[IBIS Ver]   3.2
[File Name]   sprm432.ibs
[File Rev]   1.0
[Date]   November 3, 2003
[Source]   File originated at Texas Instruments
[Copyright]   (c) 2003, Texas Instruments Inc.
[Component]   f28235zhh
[Manufacturer] Texas Instruments
[Package]
| Variable   Typ   Min   Max
R_pkg   0.08821   0.00445   0.1444
L_pkg   2.312e-09   3.373e-10   3.933e-09
C_pkg   2.855e-13   1.279e-13   4.259e-13
[Pin] signal_name   model_name   R_pin   L_pin   C_pin
B2   GPIO[30]   BC3325CFHYPU  0.09209  2.36e-09   2.324e-13
C2   GPIO[29]   BC3325CFHYPU  0.08702  2.145e-09  2.491e-13
C3   VSS   NC   0.08455  2.129e-09  2.412e-13
B1   VDD   NC   0.1237   3.291e-09  3.802e-13
C1   GPIO[0]   BC3350AFHYPU  0.103   2.673e-09  3.339e-13
D3   GPIO[1]   BC3350AFHYPU  0.07884  2.005e-09  2.389e-13
D2   GPIO[2]   BC3350AFHYPU  0.07849  1.946e-09  2.548e-13
D1   VSS   NC   0.09972  2.597e-09  2.918e-13
F5   VDDIO   NC   0.1392   3.811e-09  4.225e-13
E4   GPIO[3]   BC3350AFHYPU  0.1002   2.62e-09   3.512e-13
E2   GPIO[4]   BC3350AFHYPU  0.07253  1.807e-09  2.304e-13
E3   GPIO[5]   BC3350AFHYPU  0.07152  1.838e-09  2.399e-13
E1   GPIO[6]   BC3350AFHYPU  0.09207  2.431e-09  2.756e-13
F4   VSS   NC   0.09478  2.501e-09  3.059e-13
F3   VDD   NC   0.06871  1.775e-09  2.4e-13
F2   GPIO[7]   BC3350AFHYPU  0.06839  1.711e-09  2.218e-13
F1   GPIO[8]   BC3350AFHYPU  0.09079  2.383e-09  2.69e-13
G5   GPIO[9]   BC3350AFHYPU  0.1124   3.004e-09  3.787e-13
G4   GPIO[10]   BC3350AFHYPU  0.09241  2.449e-09  3.276e-13
G2   GPIO[11]   BC3350AFHYPU  0.06703  1.677e-09  2.109e-13
G3   GPIO[12]   BC3350AFHYPU  0.06663  1.72e-09   2.244e-13
G1   VSS   NC   0.08649  2.3e-09   3.064e-13
H1   VDD   NC   0.08687  2.308e-09  3.051e-13
H3   GPIO[13]   BC3350AFHYPU  0.0675   1.739e-09  2.278e-13
H2   GPIO[14]   BC3350AFHYPU  0.06857  1.71e-09   2.172e-13
H4   GPIO[15]   BC3350AFHYPU  0.0958   2.514e-09  3.319e-13
H5   GPIO[16]   BC3350AFHYPU  0.1148   3.076e-09  3.819e-13
J1   GPIO[17]   BC3350AFHYPU  0.09444  2.462e-09  2.835e-13
J2   VDD   NC   0.07272  1.804e-09  2.338e-13
J3   VSS   NC   0.07371  1.889e-09  2.436e-13
J4   VDD1A18   NC   0.09822  2.576e-09  3.054e-13
K1   VSS1AGND   NC   0.09654  2.518e-09  2.844e-13
K3   VSSA2   NC   0.07688  1.955e-09  2.515e-13
K2   VDDA2   NC   0.07656  1.898e-09  2.333e-13
K4   ADCINA[7]   NC   0.1045   2.711e-09  3.594e-13
J5   ADCINA[6]   NC   0.1444   3.933e-09  4.259e-13
L1   ADCINA[5]   NC   0.1023   2.666e-09  2.93e-13
L2   ADCINA[4]   NC   0.08196  2.025e-09  2.536e-13
L3   ADCINA[3]   NC   0.08003  2.035e-09  2.292e-13
M1   ADCINA[2]   NC   0.1022   2.66e-09   3.169e-13
N1   ADCINA[1]   NC   0.1206   3.247e-09  3.719e-13
M3   ADCINA[0]   NC   0.08199  2.072e-09  2.38e-13
M2   ADCLO   NC   0.08514  2.104e-09  2.563e-13
P1   VSSAIO   NC   0.1272   3.432e-09  3.17e-13
N2   VDDAIO   NC   0.09249  2.375e-09  2.344e-13
P2   ADCINB[0]   NC   0.1091   2.835e-09  3.24e-13
N3   ADCINB[1]   NC   0.0847   2.1e-09   2.977e-13
P3   ADCINB[2]   NC   0.1058   2.786e-09  3.224e-13
L4   ADCINB[3]   NC   0.1017   2.696e-09  3.056e-13
M4   ADCINB[4]   NC   0.07819  1.991e-09  2.576e-13
N4   ADCINB[5]   NC   0.07522  1.886e-09  2.531e-13
P4   ADCINB[6]   NC   0.09848  2.623e-09  3.028e-13
K5   ADCINB[7]   NC   0.1128   3.022e-09  3.435e-13
L5   ADCREFIN   NC   0.09136  2.382e-09  3.006e-13
N5   ADCREFM   NC   0.06842  1.716e-09  2.385e-13
P5   ADCREFP   NC   0.09175  2.499e-09  2.855e-13
M5   ADCRESEXT   NC   0.05893  1.5e-09   2.17e-13
K6   VSS2AGND   NC   0.1035   2.805e-09  3.409e-13
M6   VDD2A18   NC   0.06207  1.604e-09  2.311e-13
P6   VSS   NC   0.09133  2.468e-09  2.967e-13
N6   VDD   NC   0.06341  1.612e-09  2.156e-13
L6   GPIO[18]   BC3350AFHYPU  0.08399  2.26e-09   3.049e-13
K7   GPIO[19]   BC3350AFHYPU  0.1038   2.828e-09  3.985e-13
L7   GPIO[20]   BC3350AFHYPU  0.08372  2.239e-09  3.16e-13
P7   GPIO[21]   BC3350AFHYPU  0.0865   2.353e-09  2.75e-13
N7   GPIO[22]   BC3350AFHYPU  0.06169  1.56e-09   2.049e-13
M7   GPIO[23]   BC3350AFHYPU  0.06268  1.695e-09  2.38e-13
M8   GPIO[24]   BC3350AFHYPU  0.06259  1.694e-09  2.398e-13
N8   GPIO[25]   BC3350AFHYPU  0.0611   1.546e-09  2.12e-13
P8   VSS   NC   0.08825  2.433e-09  2.701e-13
L8   VDDIO   NC   0.08293  2.235e-09  3.129e-13
K8   GPIO[26]   BC3350AFHYPU  0.102   2.793e-09  3.815e-13
L9   GPIO[27]   BC3350AFHYPU  0.0859   2.316e-09  3.071e-13
N9   GPIO[32]   BC3350AFHYPU  0.06134  1.562e-09  2.256e-13
P9   GPIO[33]   BC3350AFHYPU  0.08678  2.402e-09  2.814e-13
M9   TDI   IC33FFSHYPU   0.05751  1.488e-09  2.185e-13
K9   TDO   OC3325CF   0.1051   2.874e-09  3.416e-13
M10   TRSTN   IC33FFSHYPD   0.06466  1.77e-09   2.525e-13
P10   TMS   IC33FFSHYPU   0.09255  2.499e-09  2.906e-13
N10   VSS   NC   0.06746  1.702e-09  2.398e-13
L10   XRSN   BC3350BFODHYPU 0.09217  2.446e-09  3.236e-13
K10   TEST1   NC   0.1143   3.12e-09   3.69e-13
P11   TEST2   NC   0.09684  2.574e-09  2.997e-13
N11   VSS   NC   0.07403  1.857e-09  2.454e-13
M11   VDD3VFL   NC   0.07441  1.903e-09  2.389e-13
L11   EMU0   BC3325CFHYPU  0.104   2.76e-09   3.07e-13
P12   EMU1   BC3325CFHYPU  0.103   2.706e-09  3.157e-13
N12   TCK   IC33FFSHYPU   0.08258  2.052e-09  2.669e-13
P13   GPIO[48]   BC3325CFHYPU  0.1083   2.856e-09  2.829e-13
N13   GPIO[49]   BC3325CFHYPU  0.09197  2.37e-09   2.499e-13
P14   GPIO[50]   BC3325CFHYPU  0.1255   3.388e-09  3.392e-13
M13   GPIO[51]   BC3325CFHYPU  0.08237  2.039e-09  2.548e-13
M12   VSS   NC   0.08225  2.075e-09  2.456e-13
N14   VDDIO   NC   0.1201   3.231e-09  3.81e-13
M14   GPIO[52]   BC3325CFHYPU  0.09891  2.59e-09   3.294e-13
L12   GPIO[53]   BC3325CFHYPU  0.07898  2.006e-09  2.447e-13
L13   GPIO[54]   BC3325CFHYPU  0.07487  1.867e-09  2.444e-13
L14   GPIO[55]   BC3325CFHYPU  0.09893  2.587e-09  2.886e-13
J10   VSS   NC   0.1386   3.798e-09  4.176e-13
K11   GPIO[56]   BC3325CFHYPU   0.09954  2.607e-09  3.482e-13
K13   GPIO[57]   BC3325CFHYPU  0.0709   1.771e-09  2.325e-13
K12   GPIO[58]   BC3325CFHYPU  0.07034  1.811e-09  2.401e-13
K14   VDD   NC   0.09406  2.475e-09  2.775e-13
J11   X2   NC   0.09311  2.447e-09  3.027e-13
J12   VSS   NC   0.0707   1.815e-09  2.418e-13
J13   X1   NC   0.06707  1.681e-09  2.219e-13
J14   XCLKIN   IC33FFSHY   0.09108  2.388e-09  2.791e-13
H10   VSS   NC   0.1139   3.036e-09  3.844e-13
H11   VDDIO   NC   0.09328  2.466e-09  3.308e-13
H13   VSS   NC   0.06503  1.629e-09  2.144e-13
H12   VDD   NC   0.06577  1.702e-09  2.25e-13
H14   GPIO[59]   BC3325CFHYPU  0.08639  2.297e-09  3.03e-13
G14   GPIO[60]   BC3325CFHYPU  0.0873   2.319e-09  3.041e-13
G12   GPIO[61]   BC3325CFHYPU  0.06918  1.777e-09  2.274e-13
G13   GPIO[62]   BC3325CFHYPU  0.06778  1.692e-09  2.146e-13
G11   GPIO[63]   BC3325CFHYPU  0.09314  2.459e-09  3.346e-13
G10   GPIO[64]   BC3325CFHYPU  0.1138   3.052e-09  3.802e-13
F14   GPIO[65]   BC3325CFHYPU  0.09404  2.462e-09  2.798e-13
F13   VDD   NC   0.06786  1.696e-09  2.218e-13
F12   VSS   NC   0.07232  1.856e-09  2.474e-13
F11   GPIO[66]   BC3325CFHYPU  0.09426  2.507e-09  3.058e-13
E14   VSS   NC   0.09525  2.497e-09  2.91e-13
E12   VDDIO   NC   0.07626  1.938e-09  2.582e-13
E13   GPIO[67]   BC3325CFHYPU  0.07579  1.878e-09  2.366e-13
E11   GPIO[68]   BC3325CFHYPU  0.1028   2.672e-09  3.561e-13
F10   GPIO[69]   BC3325CFHYPU  0.1414   3.864e-09  4.252e-13
D14   VSS   NC   0.1035   2.69e-09   2.981e-13
D13   VDD   NC   0.07795  1.936e-09  2.479e-13
D12   GPIO[70]   BC3325CFHYPU  0.08151  2.062e-09  2.503e-13
C14   GPIO[71]   BC3325CFHYPU  0.1046   2.725e-09  3.442e-13
B14   GPIO[72]   BC3325CFHYPU  0.1242   3.313e-09  3.855e-13
C12   GPIO[73]   BC3325CFHYPU  0.08905  2.226e-09  2.563e-13
C13   GPIO[74]   BC3325CFHYPU  0.0903   2.216e-09  2.631e-13
A14   GPIO[75]   BC3325CFHYPU  0.1281   3.455e-09  3.132e-13
B13   GPIO[76]   BC3325CFHYPU  0.09387  2.397e-09  2.377e-13
A13   GPIO[77]   BC3325CFHYPU  0.1042   2.726e-09  3.249e-13
B12   GPIO[78]   BC3325CFHYPU  0.00445  3.373e-10  1.279e-13
A12   GPIO[79]   BC3325CFHYPU  0.1012   2.679e-09  3.184e-13
D11   GPIO[38]   BC3325CFHYPU  0.09979  2.649e-09  3.147e-13
C11   XCLKOUT   BC3325CF   0.07303  1.881e-09  2.526e-13
B11   VDD   NC   0.07161  1.807e-09  2.388e-13
A11   VSS   NC   0.09603  2.567e-09  2.922e-13
E10   GPIO[28]   BC3325CFHYPU  0.1156   3.087e-09  3.455e-13
D10   GPIO[34]   BC3350AFHYPU  0.09186  2.405e-09  2.985e-13
B10   VDDIO   NC   0.06885  1.731e-09  2.29e-13
A10   VSS   NC   0.09485  2.561e-09  2.856e-13
C10   GPIO[36]   BC3325CFHYPU  0.063988 1.613e-09  2.243e-13
E9   VDD   NC   0.1082   2.906e-09  3.452e-13
C9   VSS   NC   0.06274  1.614e-09  2.346e-13
A9   GPIO[35]   BC3325CFHYPU  0.09338  2.506e-09  3.182e-13
B9   XRDN   BC3325CFHYPU  0.06408  1.62e-09   2.367e-13
D9   GPIO[37]   BC3325CFHYPU  0.08668  2.311e-09  3.397e-13
E8   VSS   NC   0.1043   2.833e-09  3.974e-13
D8   GPIO[40]   BC3325CFHYPU   0.08381  2.248e-09  3.111e-13
A8   GPIO[41]   BC3325CFHYPU  0.08698  2.367e-09  2.747e-13
B8   GPIO[42]   BC3325CFHYPU  0.06146  1.548e-09  2.203e-13
C8   VDD   NC   0.0627   1.691e-09  2.545e-13
C7   VSS   NC   0.06257  1.689e-09  2.491e-13
B7   GPIO[43]   BC3325CFHYPU  0.06157  1.552e-09  2.151e-13
A7   GPIO[44]   BC3325CFHYPU  0.08827  2.43e-09   2.835e-13
D7   GPIO[45]   BC3325CFHYPU  0.08506  2.269e-09  3.34e-13
E7   VDDIO   NC   0.1043   2.826e-09  3.994e-13
D6   VSS   NC   0.08576  2.305e-09  3.177e-13
B6   GPIO[46]   BC3325CFHYPU  0.0641   1.621e-09  2.324e-13
A6   GPIO[47]   BC3325CFHYPU  0.09005  2.472e-09  2.845e-13
C6   GPIO[80]   BC3325CFHYPU  0.06117  1.569e-09  2.29e-13
E6   GPIO[81]   BC3325CFHYPU  0.1067   2.898e-09  3.505e-13
C5   GPIO[82]   BC3325CFHYPU  0.06463  1.768e-09  2.521e-13
A5   VSS   NC   0.09355  2.521e-09  2.935e-13
B5   VDD   NC   0.06979  1.749e-09  2.589e-13
D5   GPIO[83]   BC3325CFHYPU  0.09531  2.493e-09  3.268e-13
E5   GPIO[84]   BC3325CFHYPU  0.115   3.131e-09  3.515e-13
A4   VDDIO   NC   0.101   2.662e-09  3.031e-13
B4   VSS   NC   0.07696  1.923e-09  2.515e-13
C4   GPIO[85]   BC3325CFHYPU  0.0785   1.993e-09  2.483e-13
D4   GPIO[86]   BC3325CFHYPU  0.1037   2.755e-09  3.086e-13
A3   GPIO[87]   BC3325CFHYPU  0.1053   2.763e-09  3.109e-13
B3   GPIO[39]   BC3325CFHYPU  0.08665  2.149e-09  2.561e-13
A2   GPIO[31]   BC3325CFHYPU  0.1087   2.841e-09  2.701e-13
| End of package information
|   Component BC3325CFHYPU
[Component]   BC3325CFHYPU
[Manufacturer]   Texas Instruments.
[Package]
| variable   typ   min   max
R_pkg   0.000   0.000   0.000
L_pkg   0.000H   0.000H   0.000H
C_pkg   0.000F   0.000F   0.000F
[Pin]  signal_name   model_name   R_pin   L_pin   C_pin
PAD   PAD   BC3325CFHYPU_3P3PU
| A   A   dummy
| GZ   GZ   dummy
| Y   Y   dummy
VSSS   VSSS   GND
VDDS   VDDS   POWER
[Model Selector]   BC3325CFHYPU
BC3325CFHYPU_2P5PU   cell  VDDS=2.75(TYP)  PI=0
BC3325CFHYPU_2P5PUZ   cell  VDDS=2.75(TYP)  PI=1
BC3325CFHYPU_3P3PU   cell  VDDS=3.3(TYP)  PI=0
BC3325CFHYPU_3P3PUZ   cell  VDDS=3.3(TYP)  PI=1
|   Component BC3350AFHYPU
[Component]   BC3350AFHYPU
[Manufacturer]   Texas Instruments.
[Package]
| variable   typ   min   max
R_pkg   0.000   0.000   0.000
L_pkg   0.000H   0.000H   0.000H
C_pkg   0.000F   0.000F   0.000F
[Pin]  signal_name   model_name   R_pin   L_pin   C_pin
PAD   PAD   BC3350AFHYPU_3P3PU
| A   A   dummy
| GZ   GZ   dummy
| Y   Y   dummy
VSSS   VSSS   GND
VDDS   VDDS   POWER
[Model Selector]  BC3350AFHYPU
BC3350AFHYPU_2P5PU   cell   VDDS=2.5V(typ)  PI=0
BC3350AFHYPU_2P5PUZ  cell   VDDS=2.5V(typ)  PI=1
BC3350AFHYPU_3P3PU   cell   VDDS=3.3V(typ)  PI=0
BC3350AFHYPU_3P3PUZ  cell   VDDS=3.3V(typ)  PI=1
|   Component OC3325CF
[Component]   OC3325CF
[Manufacturer]   Texas Instruments.
[Package]
| variable   typ   min   max
R_pkg   0.000   0.000   0.000
L_pkg   0.000H   0.000H   0.000H
C_pkg   0.000F   0.000F   0.000F
[Pin]  signal_name   model_name   R_pin   L_pin   C_pin
PAD   PAD   OC3325CF_3P3
| A   A   dummy
| GZ   GZ   dummy
VDDS   VDDS   POWER
VSSS   VSSS   GND
VSS   VSS   GND
[Model Selector]   OC3325CF
OC3325CF_2P5  cell VDDS=2.5V(typ)
OC3325CF_2P7  cell VDDS=2.75V(typ)
OC3325CF_3P3  cell VDDS=3.3V(typ)
|   Component IC33FFSHYPD
[Component]   IC33FFSHYPD
[Manufacturer]   Texas Instruments.
[Package]
| variable   typ   min   max
R_pkg   0.000   0.000   0.000
L_pkg   0.000H   0.000H   0.000H
C_pkg   0.000F   0.000F   0.000F
[Pin]  signal_name   model_name   R_pin   L_pin   C_pin
PAD   PAD   IC33FFSHYPD_3P3PD
| Y   Y   dummy
VSS   VSS   GND
VDDS   VDDS   POWER
[Model Selector]  IC33FFSHYPD
IC33FFSHYPD_2P7PD   cell with PI=0 and VDDS as 2.75(typ)
IC33FFSHYPD_2P7PDZ   cell with PI=1 and VDDS as 2.75(typ)
IC33FFSHYPD_3P3PD   cell with PI=0 and VDDS as 3.3(typ)
IC33FFSHYPD_3P3PDZ   cell with PI=1 and VDDS as 3.3(typ)
|   Component IC33FFSHYPU
[Component]   IC33FFSHYPU
[Manufacturer]   Texas Instruments.
[Package]
| variable   typ   min   max
R_pkg   0.000   0.000   0.000
L_pkg   0.000H   0.000H   0.000H
C_pkg   0.000F   0.000F   0.000F
[Pin]  signal_name   model_name   R_pin   L_pin   C_pin
PAD   PAD   IC33FFSHYPU_3P3PU
| Y   Y   dummy
VSS   VSS   GND
VDDS   VDDS   POWER
[Model Selector]  IC33FFSHYPU
IC33FFSHYPU_2P5PU   cell with PI=0 VDDS=2.5(typ)
IC33FFSHYPU_2P5PUZ   cell with PI=1 VDDS=2.5(typ)
IC33FFSHYPU_2P7PU   cell with PI=0 VDDS=2.7(typ)
IC33FFSHYPU_2P7PUZ   cell with PI=1 VDDS=2.7(typ)
IC33FFSHYPU_3P3PU   cell with PI=0 VDDS=3.3(typ)
IC33FFSHYPU_3P3PUZ   cell with PI=1 VDDS=3.3(typ)
|   Component BC3325CF
[Component]   BC3325CF
[Manufacturer]   Texas Instruments.
[Package]
| variable   typ   min   max
R_pkg   0.000   0.000   0.000
L_pkg   0.000H   0.000H   0.000H
C_pkg   0.000F   0.000F   0.000F
[Pin]  signal_name   model_name   R_pin   L_pin   C_pin
PAD   PAD   BC3325CF_3P3PU
| A   A   dummy
| GZ   GZ   dummy
| Y   Y   dummy
VSSS   VSSS   GND
VDDS   VDDS   POWER
[Model Selector]  BC3325CF
BC3325CF_2P5PU  cell   VDDS=2.75V(typ)
BC3325CF_3P3PU  cell   VDDS=3.30V(typ)
|   Component BC3350BFODHYPU
[Component]   BC3350BFODHYPU
[Manufacturer]   Texas Instruments.
[Package]
| variable   typ   min   max
R_pkg   0.000   0.000   0.000
L_pkg   0.000H   0.000H   0.000H
C_pkg   0.000F   0.000F   0.000F
[Pin]  signal_name   model_name   R_pin   L_pin   C_pin
PAD   PAD   BC3350BFODHYPU_3P3PU
| A   A   dummy
| GZ   GZ   dummy
| Y   Y   dummy
VSSS   VSSS   GND
VDDS   VDDS   POWER
[Model Selector]   BC3350BFODHYPU
BC3350BFODHYPU_2P5PU   cell   VDDS=2.75(TYP)
BC3350BFODHYPU_2P5PZ   cell   VDDS=2.75(TYP)
BC3350BFODHYPU_3P3PU   cell   VDDS=3.3(TYP)
BC3350BFODHYPU_3P3PZ   cell   VDDS=3.3(TYP)
|   Component IC33FFSHY
[Component]   IC33FFSHY
[Manufacturer]   Texas Instruments.
[Package]
| variable   typ   min   max
R_pkg   0.000   0.000   0.000
L_pkg   0.000H   0.000H   0.000H
C_pkg   0.000F   0.000F   0.000F
[Pin]  signal_name   model_name   R_pin   L_pin   C_pin
PAD   PAD   IC33FFSHY_3P3
| Y   Y   dummy
VSS   VSS   GND
VDDS   VDDS   POWER
[Model Selector]  IC33FFSHY
IC33FFSHY_2P5   cell with VDDS=2.5(NOM)
IC33FFSHY_2P7   cell with VDDS=2.7(NOM)
IC33FFSHY_3P3   cell with VDDS=3.3(NOM)
| Models and submodels in the file (30): BC3325CFHYPU_2P5PU (I/O), BC3325CFHYPU_2P5PUZ (I/O), BC3325CFHYPU_3P3PU (I/O), BC3325CFHYPU_3P3PUZ (I/O), BC3350AFHYPU_2P5PU (I/O), BC3350AFHYPU_2P5PUZ (I/O), BC3350AFHYPU_3P3PU (I/O), BC3350AFHYPU_3P3PUZ (I/O), OC3325CF_2P5 (3-state), OC3325CF_2P7 (3-state), OC3325CF_3P3 (3-state), IC33FFSHYPD_2P7PD (Input), IC33FFSHYPD_2P7PDZ (Input), IC33FFSHYPD_3P3PD (Input), IC33FFSHYPD_3P3PDZ (Input), IC33FFSHYPU_2P5PU (Input), IC33FFSHYPU_2P5PUZ (Input), IC33FFSHYPU_2P7PU (Input), IC33FFSHYPU_2P7PUZ (Input), IC33FFSHYPU_3P3PU (Input), IC33FFSHYPU_3P3PUZ (Input), BC3325CF_2P5PU (I/O), BC3325CF_3P3PU (I/O), BC3350BFODHYPU_2P5PU (I/O_open_drain), BC3350BFODHYPU_2P5PZ (I/O_open_drain), BC3350BFODHYPU_3P3PU (I/O_open_drain), BC3350BFODHYPU_3P3PZ (I/O_open_drain), IC33FFSHY_2P5 (Input), IC33FFSHY_2P7 (Input), IC33FFSHY_3P3 (Input)
